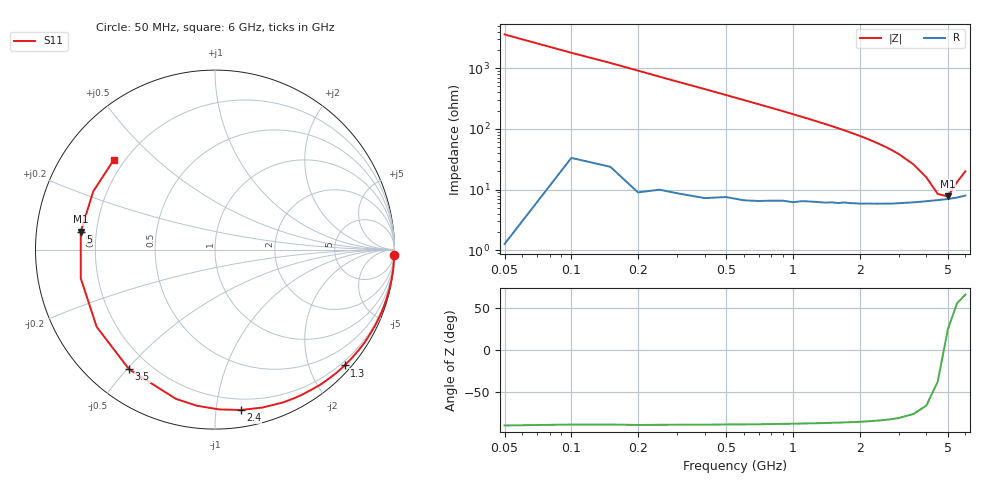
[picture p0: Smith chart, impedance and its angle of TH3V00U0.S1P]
! SIEMENS Discrete & RF Semiconductors
! BAS70
! Si Schottky Diode in SOT23
! VR = 3 V
! S-Parameters:  February  1997
# GHz  S  MA  R  50
!  f  S11
! GHz  MAG  ANG
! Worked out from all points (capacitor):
!   34 points, 50 MHz to 6 GHz, reference 50 ohm
!   read as one part to ground: C = 889 fF near 50 MHz
!   lowest |Z| = 7.75 ohm at 5 GHz (marker M1)
!   series resonance near 4.808 GHz, so ESL is about 1.2 nH
!   S11 on the Smith chart (normalised r, x): 50 MHz: 0, -72; 1.3 GHz: 0.13, -2.61; 2.4 GHz: 0.12, -1.17; 3.5 GHz: 0.12, -0.51; 5 GHz: 0.14, +0.07; 6 GHz: 0.16, +0.37
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0.05  1 -1.6
0.2  0.9989 -6.3
0.3  0.9976 -9.5
0.4  0.9965 -12.6
0.6  0.9927 -19.0
0.7  0.9904 -22.2
0.8  0.9873 -25.4
0.9  0.984 -28.6
1  0.9813 -31.9
1.1  0.9766 -35.1
1.2  0.9727 -38.4
1.3  0.9686 -41.8
1.4  0.9645 -45.1
1.6  0.9547 -51.9
1.8  0.9431 -58.9
1.9  0.9376 -62.4
2  0.9321 -66.0
2.2  0.9188 -73.3
2.4  0.9051 -80.9
2.6  0.8906 -88.6
2.8  0.8759 -96.6
3  0.8597 -104.7
3.5  0.8208 -125.7
4  0.7873 -146.9
4.5  0.7647 -167.9
5  0.7543 172.4
5.5  0.752 154.5
6  0.7536 138.6
